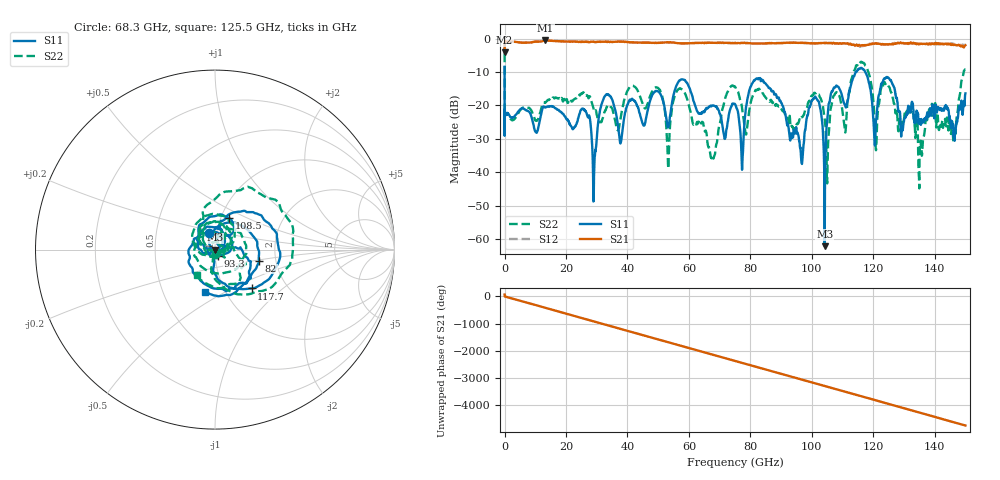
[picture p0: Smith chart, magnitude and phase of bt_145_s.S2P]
! IF Bandwidth: 10000 Hz
! Averaging: 0
! Smoothing: 0
! SourceAttenuator: 0 dB
! TestAttenuator: 0 dB
! SweepTime: 0 s
! ElectricalDelay: 0 s
# GHZ S DB R 50
! FREQ S11M S11A S21M S21A S12M S12A S22M S22A
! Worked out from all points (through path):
!   1913 points, 40 kHz to 150 GHz, reference 50 ohm
!   highest |S21| = -0.54 dB at 13.3 GHz (marker M1); lowest = -4.1 dB at 40 kHz (marker M2)
!   group delay of S21, straight-line fit = 88.1 ps
!   lowest |S11| = -62.2 dB at 104.2 GHz (marker M3), VSWR 1.00, Z = 49.9 + j0.0167 ohm
!   |S11| at or under -10 dB: 43.18 kHz to 114.3 GHz (114.3 GHz wide, 200 % of centre); 117.4 GHz to end of sweep
!   |S22| runs from -44.9 to -4.5 dB; largest |S21 - S12| = 0.14
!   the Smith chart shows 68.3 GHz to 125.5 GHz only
!   S11 on the Smith chart (normalised r, x): 68.3 GHz: 0.92, +0.17; 82 GHz: 1.63, -0.21; 93.3 GHz: 1.03, -0.07; 108.5 GHz: 1.09, +0.40; 117.7 GHz: 1.34, -0.64; 125.5 GHz: 0.80, -0.40
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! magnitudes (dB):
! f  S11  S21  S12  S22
! 40 kHz  -8.4  -4.1  -4.2  -4.5
! 86 kHz  -29.0  -1.3  -1.3  -13.0
! 13.3 GHz  -20.6  -0.5  -0.6  -19.1
! 25.1 GHz  -21.0  -0.9  -1.0  -16.4
! 29.2 GHz  -38.5  -1.0  -1.0  -21.9
! 32.9 GHz  -17.0  -0.8  -0.9  -21.5
! 37.7 GHz  -31.4  -0.9  -0.9  -24.2
! 50.1 GHz  -15.9  -1.3  -1.2  -14.9
! 68.3 GHz  -20.1  -1.2  -1.3  -35.0
! 75.1 GHz  -19.8  -1.3  -1.3  -14.5
! 77.4 GHz  -37.1  -1.3  -1.3  -21.6
! 82 GHz  -11.9  -1.5  -1.5  -15.4
! 93.3 GHz  -28.4  -1.2  -1.2  -26.5
! 100.1 GHz  -18.5  -1.5  -1.3  -17.2
! 104.2 GHz  -62.2  -1.3  -1.3  -24.1
! 108.5 GHz  -14.4  -1.5  -1.5  -16.7
! 117.7 GHz  -10.5  -1.9  -2.0  -8.3
! 120.9 GHz  -24.3  -1.4  -1.4  -33.4
! 125.1 GHz  -11.9  -1.7  -1.7  -14.3
! 125.5 GHz  -12.4  -1.6  -1.6  -15.2
! 135.5 GHz  -25.8  -1.6  -1.5  -31.7
! 150 GHz  -16.4  -2.0  -1.6  -9.2
